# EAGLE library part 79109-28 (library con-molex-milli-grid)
RECEPTACAL
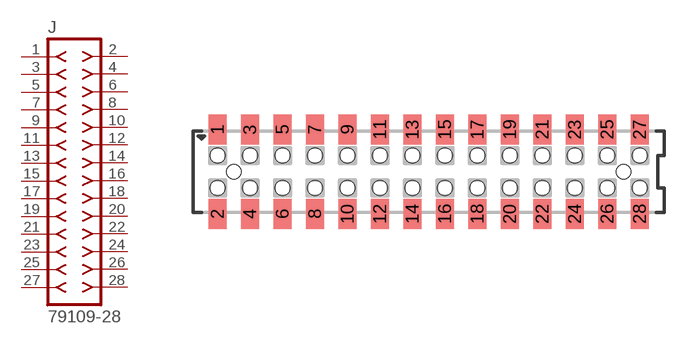
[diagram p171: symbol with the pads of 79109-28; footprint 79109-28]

Designator prefix J

## 79109-28  [79109-28]
1  1  pas
2  2  pas
3  3  pas
4  4  pas
5  5  pas
6  6  pas
7  7  pas
8  8  pas
9  9  pas
10  10  pas
11  11  pas
12  12  pas
13  13  pas
14  14  pas
15  15  pas
16  16  pas
17  17  pas
18  18  pas
19  19  pas
20  20  pas
21  21  pas
22  22  pas
23  23  pas
24  24  pas
25  25  pas
26  26  pas
27  27  pas
28  28  pas

## Footprint 79109-28 (pad centres in mm)
RECEPTACAL SMD Dual Row, Vertical, Pass-Thru
smd 1.12 x 1.83: 1 -13,2.6; 2 -13,-2.6; 3 -11,2.6; 4 -11,-2.6; 5 -9,2.6; 6 -9,-2.6; 7 -7,2.6; 8 -7,-2.6; 9 -5,2.6; 10 -5,-2.6; 11 -3,2.6; 12 -3,-2.6; 13 -1,2.6; 14 -1,-2.6; 15 1,2.6; 16 1,-2.6; 17 3,2.6; 18 3,-2.6; 19 5,2.6; 20 5,-2.6; 21 7,2.6; 22 7,-2.6; 23 9,2.6; 24 9,-2.6; 25 11,2.6; 26 11,-2.6; 27 13,2.6; 28 13,-2.6
hole 0.914 at -12,0
hole 0.914 at -13,1
hole 0.914 at -13,-1
hole 0.914 at -11,-1
hole 0.914 at -11,1
hole 0.914 at -9,-1
hole 0.914 at -9,1
hole 0.914 at 12,0
hole 0.914 at -7,1
hole 0.914 at -7,-1
hole 0.914 at -5,1
hole 0.914 at -5,-1
hole 0.914 at -3,1
hole 0.914 at -3,-1
hole 0.914 at -1,1
hole 0.914 at -1,-1
hole 0.914 at 1,-1
hole 0.914 at 1,1
hole 0.914 at 3,1
hole 0.914 at 3,-1
hole 0.914 at 5,1
hole 0.914 at 5,-1
hole 0.914 at 7,1
hole 0.914 at 7,-1
hole 0.914 at 9,-1
hole 0.914 at 9,1
hole 0.914 at 11,1
hole 0.914 at 13,1
hole 0.914 at 11,-1
hole 0.914 at 13,-1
